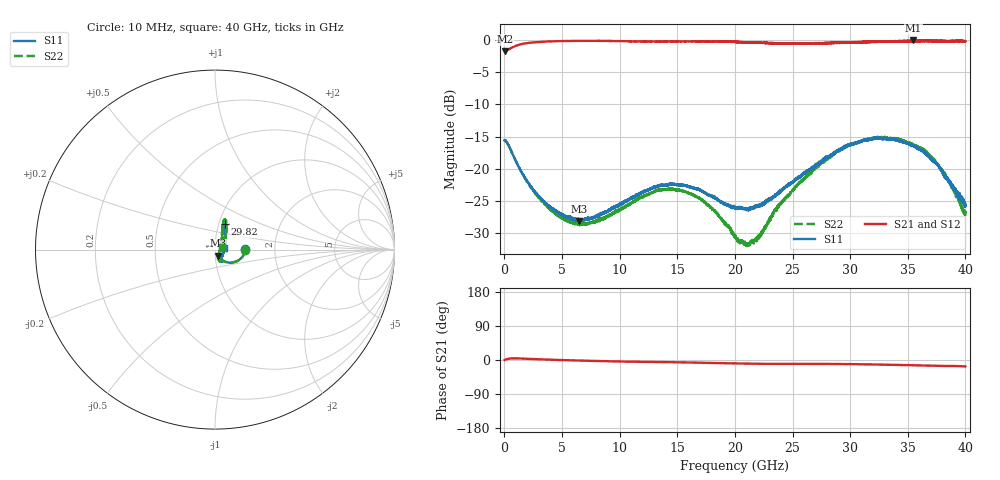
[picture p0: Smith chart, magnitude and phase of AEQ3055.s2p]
# GHZ S DB R 50.00000
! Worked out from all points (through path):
!   6401 points, 10 MHz to 40 GHz, reference 50 ohm
!   highest |S21| = -0.06 dB at 35.48 GHz (marker M1); lowest = -1.7 dB at 34.99 MHz (marker M2)
!   group delay of S21, straight-line fit = 1.26 ps
!   lowest |S11| = -28.1 dB at 6.483 GHz (marker M3), VSWR 1.08, Z = 51.8 - j3.58 ohm
!   |S11| at or under -10 dB: start of sweep to end of sweep
!   |S22| runs from -32.0 to -15.0 dB; largest |S21 - S12| = 0.014
!   S11 on the Smith chart (normalised r, x): 10 MHz: 1.40, +0.01; 29.82 GHz: 1.07, +0.31; 40 GHz: 1.11, +0.02
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0.01  -15.57 0.8  -1.69 -0.0  -1.71 0.2  -15.45 -0.3
0.03499375  -15.60 -2.0  -1.72 0.5  -1.71 0.5  -15.55 -2.2
0.8660359  -18.32 -36.4  -0.96 4.4  -0.96 4.4  -18.35 -36.2
3.027995  -24.36 -60.7  -0.29 1.8  -0.29 1.8  -24.52 -60.2
4.908775  -27.02 -65.2  -0.16 -0.1  -0.16 -0.1  -27.52 -64.8
6.483381  -28.10 -61.4  -0.12 -1.4  -0.12 -1.4  -28.38 -62.9
6.677083  -27.98 -62.2  -0.12 -1.6  -0.12 -1.6  -28.51 -62.4
8.651589  -26.72 -56.0  -0.13 -3.1  -0.13 -3.1  -27.65 -58.4
13.34417  -22.66 -57.6  -0.22 -5.3  -0.23 -5.3  -23.27 -64.3
15.23744  -22.56 -60.8  -0.22 -6.2  -0.23 -6.2  -23.28 -69.7
16.94951  -23.19 -58.6  -0.19 -7.2  -0.21 -7.2  -24.62 -71.6
20.005  -26.03 -30.2  -0.28 -9.1  -0.29 -9.1  -30.68 -45.3
21.011  -26.30 -13.5  -0.33 -9.6  -0.33 -9.6  -31.87 -16.9
21.81705  -25.73 1.6  -0.41 -9.8  -0.40 -9.8  -30.97 8.1
23.6166  -23.92 27.5  -0.49 -10.2  -0.48 -10.2  -26.15 42.7
26.67208  -19.98 55.7  -0.47 -10.2  -0.47 -10.3  -20.38 65.3
29.81505  -16.27 69.0  -0.35 -10.8  -0.37 -10.9  -16.34 71.8
33.33917  -15.43 70.1  -0.22 -12.5  -0.24 -12.4  -15.27 70.6
35.47613  -16.27 66.6  -0.06 -13.9  -0.09 -13.9  -16.14 66.9
36.53212  -17.63 61.7  -0.13 -14.7  -0.15 -14.7  -17.25 61.4
38.03174  -20.51 52.0  -0.14 -15.7  -0.12 -15.6  -20.41 54.2
40  -25.52 8.4  -0.16 -16.7  -0.18 -16.4  -27.27 16.3
